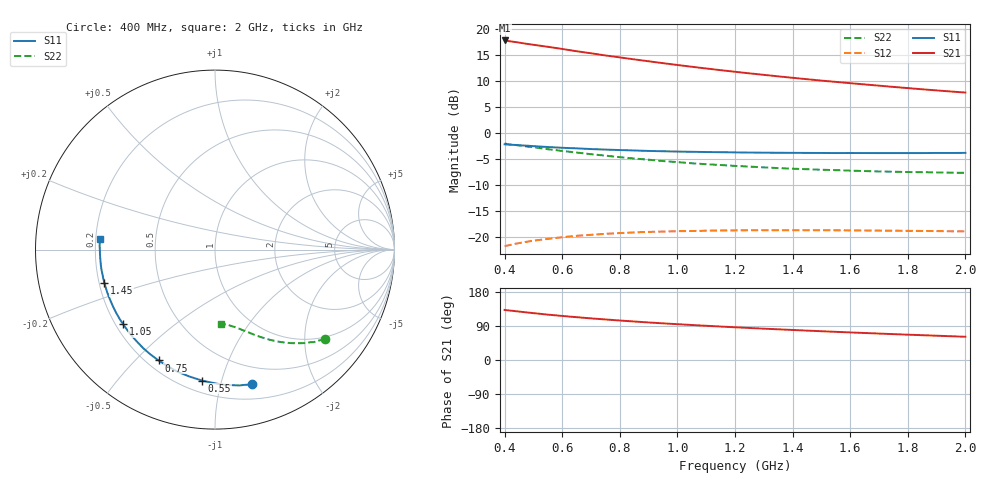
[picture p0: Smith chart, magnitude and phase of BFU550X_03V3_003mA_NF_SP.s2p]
! Filename:  P:\Prog\Test\Noise\ATS_data\Testdata_Net\BFU550X no attenuator noise\BFU550X_APG2013_44_C05_03p3V_003mA_NF_CM01_D.sf
! Date/Time: Fri 26/Jul/2013 14:37:11
! BFU550X_APG2013_44_C05_03p3V_1to10mA_NF_CM01_Bias3_R.sf
! Noise Parameter Data File
! BFU550X_APG2013_44_C05_03p3V_1to10mA_NF_CM01
! Date/time: Wed Jul 24 15:50:55 2013
! VAR V_out= 3.300000
! VAR I_out= 3.005000
! VAR V_in= 0.804700
! VAR I_in= 0.033310
! Device data file deembeded for feedlines and parallel
! Original file: \BFU550X no attenuator noise\BFU550X_APG2013_44_C05_03p3V_003mA_NF_CM01_R.sf
! Feed-files: PR005V01_100713_Feed1.s2p, PR005V01_100713_Feed2.s2p
! Parallel-file: PR005V01_100713_Par.s2p
# MHz S MA R 50
!  Freq-MHz  S11-mag  S11-arg  S21-mag  S21-arg  S12-mag  S12-arg  S22-mag  S22-arg
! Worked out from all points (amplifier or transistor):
!   37 points, 400 MHz to 2 GHz, reference 50 ohm
!   highest |S21| = 17.8 dB at 400 MHz (marker M1)
!   |S21| within 3 dB of that: start of sweep to 765.5 MHz
!   unconditionally stable (mu >= 1): nowhere
!   at 500 MHz: K = 0.20, MSG = 18.8 dB, |S12| = -20.7 dB
!   at 1.1 GHz: K = 0.41, MSG = 15.6 dB, |S12| = -18.8 dB
!   at 2 GHz: K = 0.75, MSG = 13.4 dB, |S12| = -18.9 dB
!   lowest NFmin = 0.58 dB at 420 MHz
!   S11 on the Smith chart (normalised r, x): 400 MHz: 0.33, -1.25; 550 MHz: 0.27, -0.87; 750 MHz: 0.25, -0.59; 1.05 GHz: 0.23, -0.34; 1.45 GHz: 0.22, -0.14; 2 GHz: 0.22, +0.05
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400  0.7783 -74.8  7.771 132.1  0.08158 50.2  0.7918 -39.1
420  0.7714 -77.7  7.615 130.4  0.08383 48.9  0.7764 -40.5
440  0.7665 -80.8  7.493 128.7  0.08628 47.6  0.766 -41.6
460  0.7597 -83.5  7.333 127.0  0.0883 46.2  0.7541 -43.1
500  0.7476 -89.0  7.063 123.7  0.09215 43.8  0.73 -45.5
550  0.7336 -95.6  6.755 119.8  0.09585 40.9  0.6988 -48.3
600  0.7212 -101.5  6.438 116.3  0.09947 38.5  0.6727 -50.8
650  0.7121 -106.9  6.12 113.0  0.1026 36.2  0.6492 -53.0
700  0.7011 -112.3  5.85 109.8  0.1049 34.1  0.6254 -55.2
750  0.6931 -117.0  5.576 107.0  0.1073 32.3  0.6057 -57.0
800  0.6858 -121.7  5.341 104.2  0.109 30.6  0.5858 -58.9
850  0.6795 -126.0  5.111 101.6  0.1106 29.0  0.5689 -60.5
900  0.6725 -130.1  4.9 99.1  0.1119 27.6  0.5535 -62.0
950  0.668 -133.9  4.7 96.7  0.1127 26.2  0.5375 -63.7
1050  0.6597 -140.9  4.34 92.3  0.1141 24.0  0.5118 -66.4
1200  0.6511 -150.3  3.885 86.3  0.1157 21.2  0.4827 -69.9
1300  0.6474 -155.8  3.629 82.7  0.1161 19.7  0.4671 -72.1
1450  0.6437 -163.3  3.294 77.6  0.1162 17.9  0.4485 -75.1
1500  0.6429 -165.7  3.194 75.9  0.1161 17.3  0.4434 -76.1
1600  0.6423 -170.1  3.017 72.8  0.1157 16.5  0.4347 -78.0
1750  0.6412 -176.3  2.777 68.3  0.1149 15.6  0.4243 -80.7
2000  0.6442 174.6  2.45 61.4  0.1132 14.9  0.4143 -85.0
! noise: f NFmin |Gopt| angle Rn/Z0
400  0.6049  0.3324  31.42  0.1476
460  0.5928  0.3225  46.01  0.1173
600  0.688  0.3263  46.79  0.146
800  0.6907  0.344  71.97  0.1165
1000  0.7489  0.3594  89.58  0.1041
1200  0.7642  0.3739  106.4  0.0936
1400  0.8351  0.4111  118.4  0.0867
1600  0.7981  0.4431  133.6  0.0625
1800  0.8895  0.4791  148.5  0.0462
2000  0.913  0.5112  157.5  0.0421
